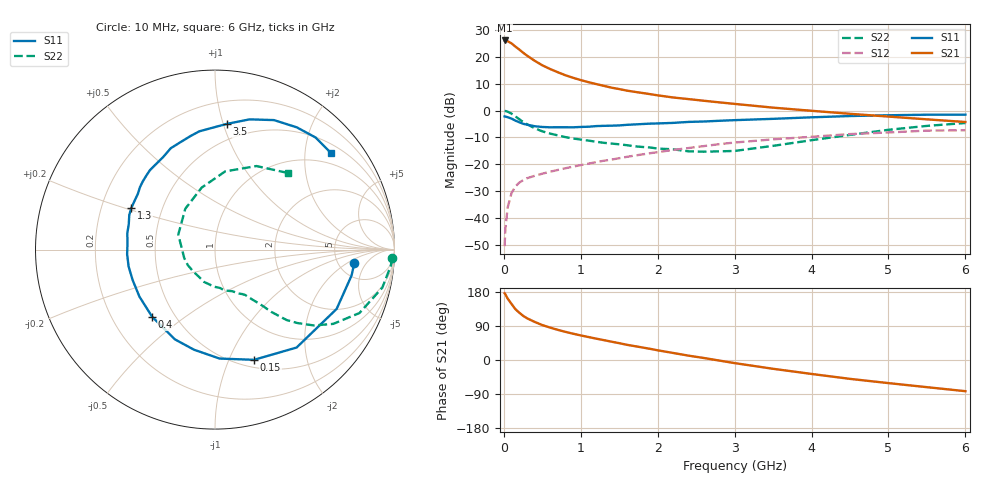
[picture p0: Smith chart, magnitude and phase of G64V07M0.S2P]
! SIEMENS Small Signal Semiconductors
! BFG193
! Si NPN RF Bipolar Junction Transistor in SOT223
! VCE = 4 V  IC = 7 mA
! Common Emitter S-Parameters:  August  1996
# GHz  S  MA  R  50
!  f  S11  S21  S12  S22
! GHz  MAG  ANG  MAG  ANG  MAG  ANG  MAG  ANG
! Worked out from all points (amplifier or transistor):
!   36 points, 10 MHz to 6 GHz, reference 50 ohm
!   highest |S21| = 26.1 dB at 10 MHz (marker M1)
!   |S21| within 3 dB of that: start of sweep to 183.2 MHz
!   unconditionally stable (mu >= 1): 1.004 GHz to 2.523 GHz
!   at 250 MHz: K = 0.43, MSG = 23.7 dB, |S12| = -25.9 dB
!   at 1.4 GHz: K = 1.08, MAG = 11.7 dB, |S12| = -18.2 dB
!   at 6 GHz: K = 0.87, MSG = 1.5 dB, |S12| = -7.3 dB
!   S11 on the Smith chart (normalised r, x): 10 MHz: 7.08, -2.66; 150 MHz: 0.58, -1.24; 400 MHz: 0.38, -0.38; 1.3 GHz: 0.33, +0.21; 3.5 GHz: 0.37, +1.03; 6 GHz: 0.71, +2.60
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0.01  0.7801 -5.4  20.22 176.1  0.003 87.6  0.9886 -2.7
0.02  0.7744 -10.8  20.12 173.4  0.0063 83.8  0.9835 -5.3
0.05  0.754 -26.0  19.59 161.9  0.0158 76.8  0.9562 -12.8
0.1  0.7102 -50.2  17.84 147.9  0.0292 67.8  0.8791 -23.7
0.15  0.6515 -70.5  15.55 134.2  0.0387 58.4  0.7785 -32.1
0.2  0.6076 -87.6  13.73 125.0  0.0456 53.9  0.6944 -37.5
0.25  0.5698 -101.9  11.99 116.7  0.0506 49.4  0.615 -41.7
0.3  0.5477 -114.1  10.58 110.3  0.0551 47.4  0.5604 -44.5
0.4  0.5125 -133.1  8.485 100.6  0.0611 45.4  0.4699 -47.8
0.5  0.4959 -148.1  6.972 92.1  0.067 43.8  0.4117 -49.7
0.6  0.4893 -159.8  5.963 85.6  0.0728 44.2  0.3746 -51.5
0.7  0.4904 -168.9  5.189 79.6  0.0785 44.4  0.3461 -53.3
0.9  0.4889 175.9  4.085 69.4  0.0907 44.4  0.3031 -56.4
1.1  0.5014 163.3  3.383 60.6  0.1031 44.7  0.2766 -62.1
1.3  0.5209 153.4  2.89 52.4  0.1168 43.8  0.2516 -67.2
1.6  0.544 140.2  2.355 40.1  0.138 41.3  0.2272 -78.7
2.2  0.5908 119.3  1.757 18.6  0.1853 33.7  0.1904 -108.5
2.8  0.6467 102.3  1.425 -1.5  0.2376 23.3  0.1744 -150.1
3.5  0.7032 84.7  1.136 -23.2  0.292 8.0  0.221 157.8
4.5  0.7929 65.5  0.872 -49.8  0.3657 -12.1  0.3533 102.1
5.5  0.8391 48.1  0.688 -71.7  0.4244 -37.2  0.5198 63.6
6  0.841 39.7  0.614 -82.3  0.4316 -51.6  0.588 46.6
